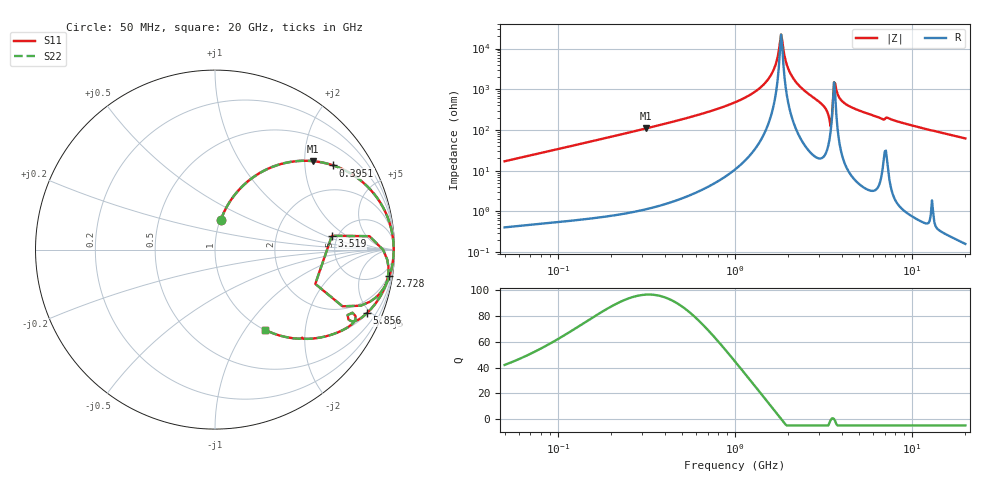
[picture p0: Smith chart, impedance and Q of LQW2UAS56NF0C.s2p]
!Murata Part Number: LQW2UAS56NF0C
!These Parameters are Measured in Series Mode Connection
!  o--[Z]--o
!Port1  Port2
!  o-------o
!Freq. Start=50[MHz] Stop=20[GHz], 401[Steps]
# Hz S RI R 50
!Freq.(Hz) S11(Real) S11(Imag) S21(Real) S21(Imag) S12(Real) S12(Imag) S22(Real) S22(Imag)
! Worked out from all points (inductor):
!   401 points, 50 MHz to 20 GHz, reference 50 ohm
!   read as one part in series: L = 54 nH near 51.52 MHz
!   highest Q = 96.7 at 315.6 MHz (marker M1), where L = 55.2 nH
!   self-resonance near 1.821 GHz
!   S11 on the Smith chart (normalised r, x): 50 MHz: 1.01, +0.34; 395.1 MHz: 1.03, +2.79; 2.728 GHz: 2, -13; 3.519 GHz: 4.47, +1.20; 5.856 GHz: 1.06, -4.74; 20 GHz: 1.00, -1.24
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5e7  0.0319 0.1642  0.9681 -0.1642  0.9681 -0.1642  0.0319 0.1642
1.364002e8  0.1798 0.3772  0.8202 -0.3772  0.8202 -0.3772  0.1798 0.3772
3.155756e8  0.5445 0.4929  0.4555 -0.4929  0.4555 -0.4929  0.5445 0.4929
3.721004e8  0.6289 0.4779  0.3711 -0.4779  0.3711 -0.4779  0.6289 0.4779
3.95076e8  0.6585 0.469  0.3415 -0.469  0.3415 -0.469  0.6585 0.469
1e9  0.9539 0.1988  0.0461 -0.1988  0.0461 -0.1988  0.9539 0.1988
1.289994e9  0.9823 0.1141  0.0177 -0.1141  0.0177 -0.1141  0.9823 0.1141
1.521052e9  0.992 0.0599  0.00804 -0.0599  0.00804 -0.0599  0.992 0.0599
1.664083e9  0.9946 0.0303  0.00535 -0.0303  0.00535 -0.0303  0.9946 0.0303
1.820564e9  0.9955 0.000591  0.00445 -0.000591  0.00445 -0.000591  0.9955 0.000591
2.083303e9  0.9934 -0.0449  0.00659 0.0449  0.00659 0.0449  0.9934 -0.0449
2.728004e9  0.9721 -0.1467  0.0279 0.1467  0.0279 0.1467  0.9721 -0.1467
3.216634e9  0.912 -0.2513  0.088 0.2513  0.088 0.2513  0.912 -0.2513
3.415248e9  0.7103 -0.3158  0.2897 0.3158  0.2897 0.3158  0.7103 -0.3158
3.519108e9  0.6512 0.0769  0.3488 -0.0769  0.3488 -0.0769  0.6512 0.0769
3.626126e9  0.9371 -0.00154  0.0629 0.00154  0.0629 0.00154  0.9371 -0.00154
3.736399e9  0.9661 -0.0951  0.0339 0.0951  0.0339 0.0951  0.9661 -0.0951
4.149438e9  0.9475 -0.2065  0.0525 0.2065  0.0525 0.2065  0.9475 -0.2065
5.856089e9  0.8456 -0.3546  0.1544 0.3546  0.1544 0.3546  0.8456 -0.3546
7.442007e9  0.7755 -0.4015  0.2245 0.4015  0.2245 0.4015  0.7755 -0.4015
1.166392e10  0.5419 -0.4958  0.4581 0.4958  0.4581 0.4958  0.5419 -0.4958
2e10  0.278 -0.4467  0.722 0.4467  0.722 0.4467  0.278 -0.4467
